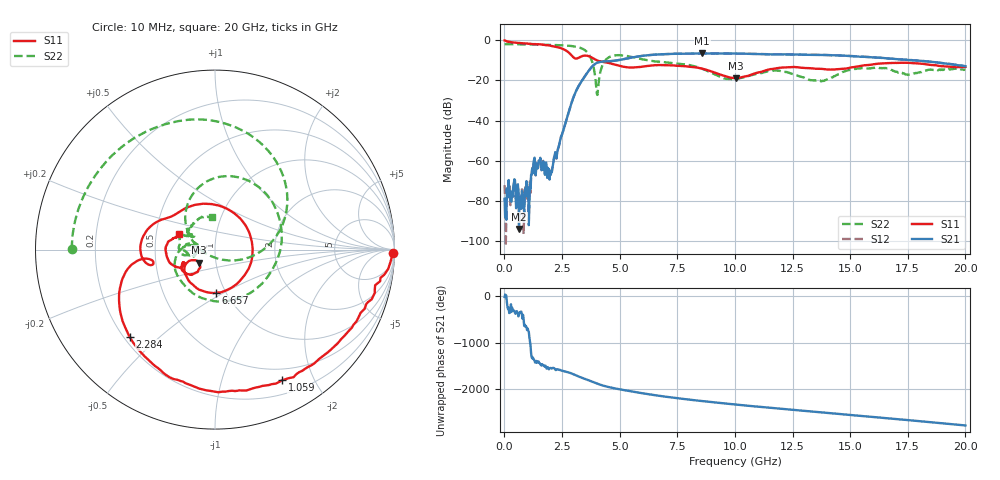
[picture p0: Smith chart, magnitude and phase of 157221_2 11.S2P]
!  2-Port S-parameters saved by WinCal
! VAR MeasName=S-Parameters (CALIBRATED_DATA) read from VNA (N5242A)
! VAR MeasDate=2015-5-26 16:47:54
! VAR NAME=157221_2 11
! VAR FILENAME=157221_2 11.S2P
! VAR DATE=2015-5-26 16:47:54
! VAR PHYS_PORTS=1,2
# Hz S DB R 50
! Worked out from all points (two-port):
!   801 points, 10 MHz to 20 GHz, reference 50 ohm
!   highest |S21| = -6.55 dB at 8.581 GHz (marker M1); lowest = -93.9 dB at 634.7 MHz (marker M2)
!   |S21| within 3 dB of the highest: 5.109 GHz to 17.2 GHz (12.09 GHz wide, 108 % of centre)
!   lowest |S11| = -18.9 dB at 10.05 GHz (marker M3), VSWR 1.26, Z = 41.5 - j6.05 ohm
!   |S11| at or under -10 dB: 4.018 GHz to end of sweep
!   |S22| runs from -27.2 to -2.0 dB; largest |S21 - S12| = 0.0093
!   S11 on the Smith chart (normalised r, x): 10 MHz: 36, -80; 1.059 GHz: 0.36, -1.58; 2.284 GHz: 0.22, -0.40; 6.657 GHz: 0.90, -0.46; 20 GHz: 0.66, +0.12
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1e7  -0.08 -1.2  -78.98 -14.2  -72.15 129.9  -1.96 179.8
6.346875e8  -1.36 -39.5  -93.92 4.7  -83.38 55.3  -2.00 164.6
1.059475e9  -1.75 -62.8  -92.07 -44.4  -90.32 98.9  -2.06 154.1
1.30935e9  -1.91 -75.9  -58.47 53.3  -58.70 53.3  -2.11 147.7
1.959025e9  -2.65 -114.3  -69.37 -110.2  -68.57 -115.4  -2.27 129.3
2.283862e9  -3.35 -134.2  -56.60 -129.5  -56.43 -129.5  -2.39 118.5
3.358325e9  -7.95 -171.1  -20.24 45.4  -20.20 45.0  -4.06 62.0
3.733138e9  -8.25 161.7  -14.07 -23.8  -14.07 -24.2  -8.43 16.8
4.032988e9  -10.07 145.2  -11.16 -82.5  -11.17 -82.8  -27.23 -128.1
4.632688e9  -11.58 103.9  -10.39 -167.5  -10.38 -167.8  -7.95 89.3
5.732138e9  -13.41 -21.5  -8.18 91.9  -8.17 91.4  -8.78 -0.3
6.656675e9  -12.37 -89.2  -7.05 20.0  -7.04 19.8  -10.60 -75.6
6.681662e9  -12.35 -90.4  -7.04 18.2  -7.02 18.0  -10.62 -77.3
8.580712e9  -14.11 -149.7  -6.55 -98.0  -6.55 -98.1  -14.20 -179.1
1.0005e10  -18.81 -141.7  -6.61 -171.2  -6.61 -171.7  -19.42 -171.2
1.005498e10  -18.89 -140.7  -6.62 -173.7  -6.62 -174.2  -19.32 -169.7
1.177911e10  -14.02 -136.1  -7.02 106.8  -6.96 106.0  -15.01 176.6
1.335332e10  -13.95 -156.0  -7.26 36.9  -7.20 36.5  -19.93 164.9
1.530235e10  -13.10 -152.8  -8.04 -50.8  -7.94 -51.1  -14.07 -177.7
1.667666e10  -11.36 -171.3  -9.07 -111.8  -9.08 -112.0  -14.19 155.3
1.82009e10  -11.83 168.9  -10.35 -179.4  -10.36 -179.8  -15.41 149.4
2e10  -13.27 156.8  -12.93 96.5  -12.93 95.3  -14.78 96.1
